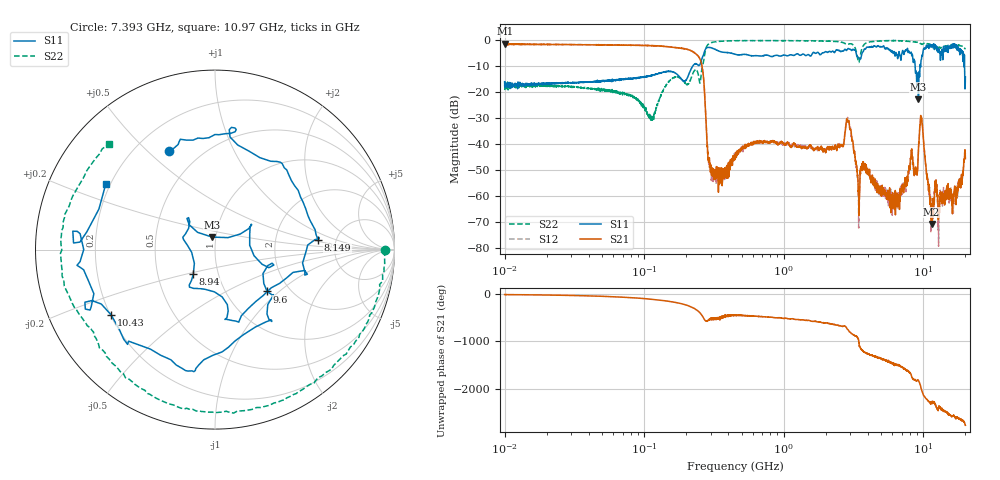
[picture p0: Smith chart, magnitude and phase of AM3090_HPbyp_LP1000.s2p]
# Hz S DB R 50
!freq MagS11 AngS11 MagS21 AngS21 MagS12 AngS12 MagS22 AngS22
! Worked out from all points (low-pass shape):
!   3201 points, 10 MHz to 20 GHz, reference 50 ohm
!   highest |S21| = -1.44 dB at 10.05 MHz (marker M1); lowest = -70.8 dB at 11.44 GHz (marker M2)
!   |S21| within 3 dB of the highest: start of sweep to 221.8 MHz
!   lowest |S11| = -22.9 dB at 9.22 GHz (marker M3), VSWR 1.15, Z = 47.9 + j6.73 ohm
!   |S11| at or under -10 dB: start of sweep to 223.2 MHz; 8.728 GHz to 9.464 GHz (735.4 MHz wide, 8.08 % of centre); 19.73 GHz to end of sweep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
!   |S22| runs from -31.4 to -0.2 dB; largest |S21 - S12| = 0.036
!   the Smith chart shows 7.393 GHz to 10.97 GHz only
!   S11 on the Smith chart (normalised r, x): 7.393 GHz: 0.34, +0.59; 8.149 GHz: 3.63, +0.59; 8.94 GHz: 0.76, -0.22; 9.6 GHz: 1.54, -0.84; 10.43 GHz: 0.20, -0.28; 10.97 GHz: 0.18, +0.27
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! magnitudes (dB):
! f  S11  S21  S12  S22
! 10 MHz  -16.1  -1.6  -1.6  -17.8
! 10.05 MHz  -16.7  -1.4  -1.5  -19.1
! 35.55 MHz  -16.4  -1.9  -1.8  -18.4
! 126.1 MHz  -12.9  -2.3  -2.3  -24.3
! 249.3 MHz  -9.7  -7.0  -7.0  -16.3
! 305.1 MHz  -3.1  -52.2  -50.4  -1.0
! 447.2 MHz  -5.5  -46.0  -44.5  -0.3
! 1.59 GHz  -5.6  -41.4  -41.5  -0.3
! 2.893 GHz  -3.3  -31.5  -30.9  -1.6
! 3.416 GHz  -6.7  -58.4  -58.2  -8.3
! 3.766 GHz  -3.6  -49.5  -48.4  -1.7
! 5.639 GHz  -3.7  -60.7  -61.8  -0.3
! 7.393 GHz  -4.3  -53.7  -55.1  -0.5
! 8.149 GHz  -4.8  -44.2  -45.6  -0.7
! 8.94 GHz  -14.8  -51.7  -52.0  -0.9
! 9.22 GHz  -22.9  -42.4  -42.4  -1.0
! 9.6 GHz  -8.6  -29.3  -30.1  -1.5
! 10.43 GHz  -3.3  -48.5  -48.2  -1.3
! 10.97 GHz  -3.0  -57.8  -56.7  -1.5
! 11.44 GHz  -2.8  -70.8  -64.5  -2.4
! 16.82 GHz  -2.4  -58.0  -59.7  -1.7
! 20 GHz  -14.3  -45.7  -43.6  -3.6
